| TEXAS INSTRUMENTS INCORPORATED
| Standard Linear and Logic Group
| IBIS Model of SN74ALVCH16823
| 18-BIT BUS-INTERFACE FLIP-FLOP WITH 3-STATE OUTPUTS
| This file contains package information for the following:
|  SSOP 56-pin (DL) package as [Component] ALVCH16823_DL
|  TSSOP 56-pin (DGG) package as [Component] ALVCH16823_DGG
| This device can be powered at the following Vccs:
|  3.3 volt Vcc
|  1.8 volt Vcc
|  2.5 volt Vcc
| This file provides unique models under the [Model Selector] for each Vcc.
| For operation at a specific Vcc, select the appropriate model after each
| [Model Selector] keyword.
[IBIS Ver]   3.2
[Comment char]  |_char
[File Name]   sn74alvch16823.ibs
[File Rev]   1.1 | k_die
[Date]   June 7, 2002
[Source]   Data created from TI-SPICE simulations at TI-SLL.
[Notes]   The following is an IBIS list for the ALVCH16823.
   Please contact sllibis@ti.com with questions and
   comments concerning SLL IBIS models.
   -Power clamp data has been deleted from CLIN and CEIN models
   since there is no power clamp diode for those inputs.
   -C_comp values are taken at a different test condition
   than the data sheet.
   -Non-monotonic data in ground-clamp due to bus-hold
[Disclaimer] Property of Texas Instruments Incorporated.  Unauthorized
   reproduction and/or distribution is strictly prohibited.
   This product is protected under copyright law.
   Created  2002, (C) Copyright  2002, Texas Instruments
   Incorporated, All Rights Reserved
   UNLESS THERE IS A SIGNED, WRITTEN AGREEMENT TO THE
   CONTRARY, TEXAS INSTRUMENTS (TI) IS PROVIDING THE IBIS
   MODELS  AND WITHOUT ANY WARRANTY, EXPRESSED OR
   IMPLIED.  TI assumes no liability for:
   1) the accuracy of the IBIS models provided to your
   company;
   2) the proper functioning of these IBIS Models in your
   design or for any resulting applications; or
   3) infringement of patents, copyrights or intellectual
   property rights resulting from your use of these IBIS
   models.
   TI provides IBIS Models as a service to our customers.
   You and your company shall not distribute, sell or give
   these models to anyone else without prior written
   permission from TI.
   TI reserves the right to make changes to our products or
   to discontinue any semiconductor product or service
   without notice, and advises our customers to obtain the
   latest version of relevant information to verify, before
   placing orders, that the information being relied on is
   current.
   Please be aware that your receipt and use of the IBIS
   information provided shall serve as acceptance of these
   terms and conditions.  If you do not accept these terms,
   you should return or destroy the IBIS models and any
   other accompanying information immediately.
| Component ALVCH16823_DL 56-pin SSOP
[Component]   ALVCH16823_DL
[Manufacturer]   Texas Instruments, Inc.
[Package]
|   typ   min   max
R_pkg   5.500e-02   4.800e-02   6.700e-02
L_pkg   6.539e-09   4.802e-09   9.746e-09
C_pkg   1.880e-13   7.600e-14   5.170e-13
[Pin]   signal_name   model_name   R_pin   L_pin   C_pin
1   1CLR   ALVCH16823_CLIN   6.400e-02   9.646e-09   5.130e-13
2   1OE   ALVCH16823_OEIN   5.900e-02   8.723e-09   2.700e-13
3   1Q1   ALVCH16823_OUT   5.900e-02   8.139e-09   2.230e-13
4   GND   GND   5.600e-02   7.554e-09   2.010e-13
5   1Q2   ALVCH16823_OUT   5.400e-02   6.991e-09   1.950e-13
6   1Q3   ALVCH16823_OUT   5.300e-02   6.659e-09   2.020e-13
7   VCC   POWER   5.500e-02   6.321e-09   2.070e-13
8   1Q4   ALVCH16823_OUT   5.500e-02   5.942e-09   1.330e-13
9   1Q5   ALVCH16823_OUT   5.700e-02   5.767e-09   1.320e-13
10   1Q6   ALVCH16823_OUT   5.400e-02   5.459e-09   1.210e-13
11   GND   GND   5.100e-02   5.224e-09   1.400e-13
12   1Q7   ALVCH16823_OUT   4.800e-02   5.088e-09   1.260e-13
13   1Q8   ALVCH16823_OUT   5.000e-02   5.021e-09   9.600e-14
14   1Q9   ALVCH16823_OUT   5.100e-02   4.802e-09   7.600e-14
15   2Q1   ALVCH16823_OUT   5.100e-02   4.803e-09   7.600e-14
16   2Q2   ALVCH16823_OUT   5.000e-02   5.021e-09   9.600e-14
17   2Q3   ALVCH16823_OUT   4.800e-02   5.088e-09   1.260e-13
18   GND   GND   5.100e-02   5.224e-09   1.400e-13
19   2Q4   ALVCH16823_OUT   5.400e-02   5.459e-09   1.210e-13
20   2Q5   ALVCH16823_OUT   5.700e-02   5.768e-09   1.330e-13
21   2Q6   ALVCH16823_OUT   5.500e-02   5.942e-09   1.330e-13
22   VCC   POWER   5.500e-02   6.320e-09   2.060e-13
23   2Q7   ALVCH16823_OUT   5.300e-02   6.659e-09   2.030e-13
24   2Q8   ALVCH16823_OUT   5.400e-02   6.991e-09   1.960e-13
25   GND   GND   5.600e-02   7.554e-09   2.010e-13
26   2Q9   ALVCH16823_OUT   5.900e-02   8.139e-09   2.230e-13
27   2OE   ALVCH16823_OEIN   5.900e-02   8.727e-09   2.700e-13
28   2CLR   ALVCH16823_CLIN   6.700e-02   9.746e-09   5.170e-13
29   2CLK   ALVCH16823_CKIN   6.300e-02   9.630e-09   5.110e-13
30   2CLKEN   ALVCH16823_CEIN   6.000e-02   8.751e-09   2.710e-13
31   2D9   ALVCH16823_IN   6.000e-02   8.184e-09   2.250e-13
32   GND   GND   5.600e-02   7.543e-09   2.000e-13
33   2D8   ALVCH16823_IN   5.400e-02   7.005e-09   1.960e-13
34   2D7   ALVCH16823_IN   5.600e-02   6.714e-09   2.040e-13
35   VCC   POWER   5.800e-02   6.384e-09   2.080e-13
36   2D6   ALVCH16823_IN   5.700e-02   5.976e-09   1.340e-13
37   2D5   ALVCH16823_IN   5.700e-02   5.743e-09   1.300e-13
38   2D4   ALVCH16823_IN   5.400e-02   5.468e-09   1.190e-13
39   GND   GND   5.500e-02   5.328e-09   1.420e-13
40   2D3   ALVCH16823_IN   5.200e-02   5.189e-09   1.290e-13
41   2D2   ALVCH16823_IN   5.200e-02   5.053e-09   9.600e-14
42   2D1   ALVCH16823_IN   5.100e-02   4.825e-09   7.600e-14
43   1D9   ALVCH16823_IN   5.400e-02   4.896e-09   7.800e-14
44   1D8   ALVCH16823_IN   5.200e-02   5.093e-09   9.700e-14
45   1D7   ALVCH16823_IN   5.100e-02   5.179e-09   1.280e-13
46   GND   GND   5.400e-02   5.314e-09   1.420e-13
47   1D6   ALVCH16823_IN   5.500e-02   5.511e-09   1.210e-13
48   1D5   ALVCH16823_IN   5.700e-02   5.771e-09   1.310e-13
49   1D4   ALVCH16823_IN   5.600e-02   5.957e-09   1.330e-13
50   VCC   POWER   5.500e-02   6.320e-09   2.060e-13
51   1D3   ALVCH16823_IN   5.200e-02   6.621e-09   2.000e-13
52   1D2   ALVCH16823_IN   5.300e-02   6.973e-09   1.950e-13
53   GND   GND   5.700e-02   7.571e-09   2.020e-13
54   1D1   ALVCH16823_IN   5.700e-02   8.097e-09   2.220e-13
55   1CLKEN   ALVCH16823_CEIN   5.900e-02   8.723e-09   2.710e-13
56   1CLK   ALVCH16823_CKIN   6.100e-02   9.560e-09   5.090e-13
| Component ALVCH16823_DGG 56-pin TSSOP
[Component]   ALVCH16823_DGG
[Manufacturer]   Texas Instruments, Inc.
[Package]
|   typ   min   max
R_pkg   4.500e-02   3.500e-02   6.200e-02
L_pkg   3.324e-09   2.403e-09   5.094e-09
C_pkg   5.640e-13   3.410e-13   9.140e-13
[Pin]   signal_name   model_name   R_pin   L_pin   C_pin
1   1CLR   ALVCH16823_CLIN   6.200e-02   5.094e-09   8.560e-13
2   1OE   ALVCH16823_OEIN   6.100e-02   4.621e-09   9.020e-13
3   1Q1   ALVCH16823_OUT   6.000e-02   4.316e-09   8.020e-13
4   GND   GND   5.900e-02   3.968e-09   6.980e-13
5   1Q2   ALVCH16823_OUT   5.700e-02   3.716e-09   6.490e-13
6   1Q3   ALVCH16823_OUT   4.200e-02   3.517e-09   6.520e-13
7   VCC   POWER   4.100e-02   3.160e-09   5.700e-13
8   1Q4   ALVCH16823_OUT   3.900e-02   2.981e-09   4.820e-13
9   1Q5   ALVCH16823_OUT   3.900e-02   2.809e-09   4.470e-13
10   1Q6   ALVCH16823_OUT   3.800e-02   2.715e-09   4.090e-13
11   GND   GND   4.100e-02   2.675e-09   3.910e-13
12   1Q7   ALVCH16823_OUT   3.900e-02   2.536e-09   3.660e-13
13   1Q8   ALVCH16823_OUT   3.900e-02   2.457e-09   3.480e-13
14   1Q9   ALVCH16823_OUT   3.800e-02   2.411e-09   3.530e-13
15   2Q1   ALVCH16823_OUT   3.900e-02   2.456e-09   3.550e-13
16   2Q2   ALVCH16823_OUT   3.900e-02   2.471e-09   3.490e-13
17   2Q3   ALVCH16823_OUT   4.000e-02   2.580e-09   3.700e-13
18   GND   GND   3.800e-02   2.651e-09   3.890e-13
19   2Q4   ALVCH16823_OUT   3.800e-02   2.739e-09   4.110e-13
20   2Q5   ALVCH16823_OUT   3.900e-02   2.838e-09   4.490e-13
21   2Q6   ALVCH16823_OUT   3.800e-02   2.988e-09   4.840e-13
22   VCC   POWER   3.800e-02   3.105e-09   5.640e-13
23   2Q7   ALVCH16823_OUT   4.000e-02   3.427e-09   6.380e-13
24   2Q8   ALVCH16823_OUT   5.600e-02   3.654e-09   6.410e-13
25   GND   GND   5.700e-02   3.932e-09   7.000e-13
26   2Q9   ALVCH16823_OUT   5.800e-02   4.257e-09   8.060e-13
27   2OE   ALVCH16823_OEIN   5.700e-02   4.580e-09   9.140e-13
28   2CLR   ALVCH16823_CLIN   5.900e-02   5.038e-09   8.610e-13
29   2CLK   ALVCH16823_CKIN   6.000e-02   5.058e-09   8.580e-13
30   2CLKEN   ALVCH16823_CEIN   5.600e-02   4.543e-09   9.040e-13
31   2D9   ALVCH16823_IN   5.700e-02   4.240e-09   8.030e-13
32   GND   GND   5.700e-02   3.929e-09   7.000e-13
33   2D8   ALVCH16823_IN   5.600e-02   3.616e-09   6.370e-13
34   2D7   ALVCH16823_IN   3.700e-02   3.368e-09   6.400e-13
35   VCC   POWER   3.600e-02   3.024e-09   5.630e-13
36   2D6   ALVCH16823_IN   3.500e-02   2.876e-09   4.740e-13
37   2D5   ALVCH16823_IN   3.500e-02   2.745e-09   4.440e-13
38   2D4   ALVCH16823_IN   3.700e-02   2.683e-09   4.050e-13
39   GND   GND   3.800e-02   2.603e-09   3.820e-13
40   2D3   ALVCH16823_IN   3.800e-02   2.510e-09   3.620e-13
41   2D2   ALVCH16823_IN   3.600e-02   2.412e-09   3.410e-13
42   2D1   ALVCH16823_IN   3.800e-02   2.416e-09   3.490e-13
43   1D9   ALVCH16823_IN   3.700e-02   2.403e-09   3.490e-13
44   1D8   ALVCH16823_IN   3.700e-02   2.429e-09   3.410e-13
45   1D7   ALVCH16823_IN   3.600e-02   2.482e-09   3.580e-13
46   GND   GND   3.700e-02   2.615e-09   3.810e-13
47   1D6   ALVCH16823_IN   3.500e-02   2.669e-09   4.020e-13
48   1D5   ALVCH16823_IN   3.600e-02   2.763e-09   4.420e-13
49   1D4   ALVCH16823_IN   3.600e-02   2.942e-09   4.780e-13
50   VCC   POWER   3.500e-02   3.053e-09   5.640e-13
51   1D3   ALVCH16823_IN   3.600e-02   3.409e-09   6.410e-13
52   1D2   ALVCH16823_IN   5.800e-02   3.698e-09   6.410e-13
53   GND   GND   5.900e-02   3.975e-09   6.970e-13
54   1D1   ALVCH16823_IN   6.100e-02   4.327e-09   8.020e-13
55   1CLKEN   ALVCH16823_CEIN   6.100e-02   4.624e-09   9.050e-13
56   1CLK   ALVCH16823_CKIN   6.000e-02   5.063e-09   8.580e-13
| Model ALVCH16823_CLIN
[Model Selector]   ALVCH16823_CLIN
ALVCH16823_CLIN_33   3.3 volt Vcc
ALVCH16823_CLIN_18   1.8 volt Vcc
ALVCH16823_CLIN_25   2.5 volt Vcc
| Model ALVCH16823_CEIN
[Model Selector]   ALVCH16823_CEIN
ALVCH16823_CEIN_33   3.3 volt Vcc
ALVCH16823_CEIN_18   1.8 volt Vcc
ALVCH16823_CEIN_25   2.5 volt Vcc
| Model ALVCH16823_IN
[Model Selector]   ALVCH16823_IN
ALVCH16823_IN_33   3.3 volt Vcc
ALVCH16823_IN_18   1.8 volt Vcc
ALVCH16823_IN_25   2.5 volt Vcc
| Model ALVCH16823_OEIN
[Model Selector]   ALVCH16823_OEIN
ALVCH16823_OEIN_33   3.3 volt Vcc
ALVCH16823_OEIN_18   1.8 volt Vcc
ALVCH16823_OEIN_25   2.5 volt Vcc
| Model ALVCH16823_CKIN
[Model Selector]   ALVCH16823_CKIN
ALVCH16823_CKIN_33   3.3 volt Vcc
ALVCH16823_CKIN_18   1.8 volt Vcc
ALVCH16823_CKIN_25   2.5 volt Vcc
| Model ALVCH16823_OUT
[Model Selector]   ALVCH16823_OUT
ALVCH16823_OUT_33   3.3 volt Vcc
ALVCH16823_OUT_18   1.8 volt Vcc
ALVCH16823_OUT_25   2.5 volt Vcc
| Models and submodels in the file (18): ALVCH16823_CLIN_33 (Input), ALVCH16823_CLIN_18 (Input), ALVCH16823_CLIN_25 (Input), ALVCH16823_CEIN_33 (Input), ALVCH16823_CEIN_18 (Input), ALVCH16823_CEIN_25 (Input), ALVCH16823_IN_33 (Input), ALVCH16823_IN_18 (Input), ALVCH16823_IN_25 (Input), ALVCH16823_OEIN_33 (Input), ALVCH16823_OEIN_18 (Input), ALVCH16823_OEIN_25 (Input), ALVCH16823_CKIN_33 (Input), ALVCH16823_CKIN_18 (Input), ALVCH16823_CKIN_25 (Input), ALVCH16823_OUT_33 (3-state), ALVCH16823_OUT_18 (3-state), ALVCH16823_OUT_25 (3-state)
